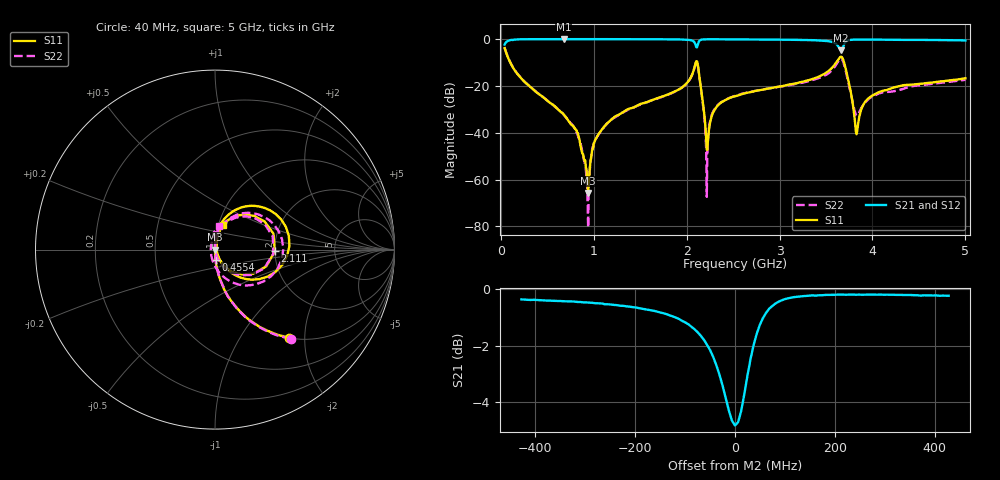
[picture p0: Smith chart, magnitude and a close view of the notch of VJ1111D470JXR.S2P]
! VJ1111D470JXR
! DATE 02/16/2022  11:09
! CAPACITORS MOUNTED IN SERIES ON 25 MIL THICK MICROSTRIP SUBSTRATE
# GHz  S  MA  R  50.00
!  FREQ  S11M  S11A  S21M  S21A  S12M  S12A  S22M  S22A
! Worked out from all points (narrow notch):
!   801 points, 40 MHz to 5 GHz, reference 50 ohm
!   highest |S21| = -0.01 dB at 678.6 MHz (marker M1); lowest = -4.8 dB at 3.661 GHz (marker M2)
!   notch at M2: 4.6 dB deep, 72 MHz wide at half that depth
!   lowest |S11| = -65.7 dB at 939 MHz (marker M3), VSWR 1.00, Z = 50 + j0.0229 ohm
!   |S11| at or under -10 dB: 100.6 MHz to 2.098 GHz (1.998 GHz wide, 182 % of centre); 2.114 GHz to 3.61 GHz (1.496 GHz wide, 52.3 % of centre); 3.694 GHz to end of sweep
!   |S22| runs from -80.6 to -3.7 dB; largest |S21 - S12| = 0.038
!   S11 on the Smith chart (normalised r, x): 40 MHz: 1.01, -1.68; 455.4 MHz: 1.00, -0.11; 2.111 GHz: 2.00, -0.04; 5 GHz: 1.05, +0.30
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0.04  0.6427 -49.8  0.7626 40.1  0.7637 40.3  0.6512 -49.7
0.1392  0.23 -77.0  0.9685 13.1  0.9786 14.9  0.2338 -75.9
0.4554  0.05715 -86.4  0.997 4.2  1.002 4.2  0.05735 -86.1
0.6786  0.02425 -87.7  0.9984 2.3  1.003 2.0  0.02393 -88.6
0.8088  0.01138 -86.4  0.9966 1.7  1.004 1.5  0.01094 -90.1
0.8708  0.00402 -79.4  0.9976 1.5  1.004 1.3  0.004469 -86.0
0.939  0.0005185 26.2  0.9964 1.2  1.003 1.1  9.376e-05 -77.3
1.001  0.006069 82.6  0.9972 1.1  1.003 0.8  0.005838 85.9
1.1126  0.01361 85.9  0.9965 0.8  1.002 0.5  0.01331 89.6
1.6954  0.05526 84.7  0.9887 -0.8  0.9958 -1.0  0.05483 84.8
1.9682  0.09915 79.8  0.9746 -2.9  0.9815 -3.1  0.09774 78.6
2.1108  0.3334 -1.6  0.6661 5.7  0.6706 5.5  0.3255 -4.2
2.2224  0.004271 34.6  0.9889 2.9  0.9953 2.7  0.003575 90.9
2.303  0.03154 86.3  0.9892 1.3  0.9952 1.1  0.03252 90.4
2.52  0.06012 85.3  0.9828 -0.1  0.9903 -0.4  0.06096 88.8
3.3508  0.1397 77.3  0.9479 -3.7  0.9548 -3.9  0.1329 77.0
3.6608  0.4186 10.8  0.5743 3.5  0.5796 3.3  0.3809 0.8
3.7228  0.1868 -51.0  0.9064 14.8  0.9134 14.6  0.1677 -70.6
3.8282  0.009273 5.9  0.9741 5.5  0.981 5.2  0.02349 -173.9
3.9398  0.05023 77.2  0.9765 2.7  0.9834 2.5  0.04839 110.1
4.1754  0.08456 79.4  0.9688 0.3  0.9747 0.2  0.07465 92.6
5  0.1453 72.6  0.9355 -3.0  0.9427 -3.2  0.135 80.9
